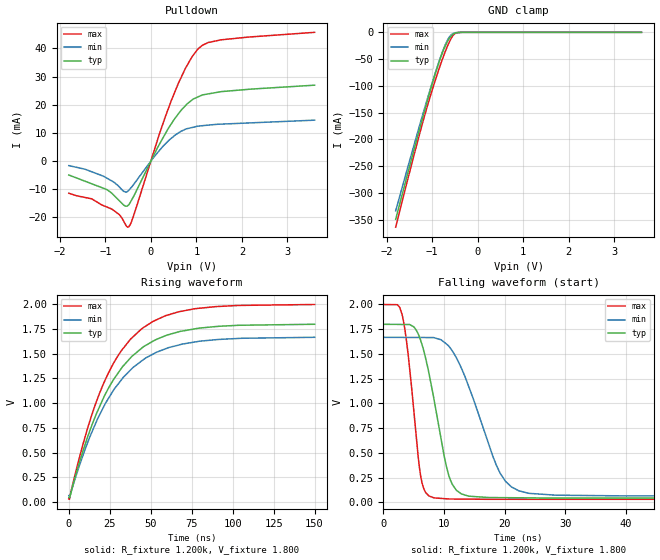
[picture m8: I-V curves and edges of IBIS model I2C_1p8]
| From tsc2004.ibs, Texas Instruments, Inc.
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| Model 1.8 V I2C
[Model]   I2C_1p8
Model_type   I/O_open_drain
Polarity   Non-Inverting
Enable   Active-Low
Vinl = 0.54
Vinh = 1.26
Vmeas = 0.9
Vref = 0.9
Cref = 15pF
Rref = 1200
|   typ   min   max
|   (nom PVT)   (Fast PVT)   (slow PVT)
|   Output High
C_comp   1.38702E-11   1.38702E-11   1.38702E-11
|   Output Low
|C_comp   1.34302E-11   1.32458E-11   1.39342E-11
| Where   nom PVT is  Nominal Process, 3.3V, 25C
|   Fast PVT is Strong Process, 3.6V, -40C
|   Slow PVT is Weak Process, 3.0V, 85C
|C_comp - from L-C Tank method, L = 1nH, peak frequency ~ 1.35GHz
[Model Spec]   | power 1.8, 1.65. 2 V
Vinl   0.54   0.495   0.6
Vinh   1.26   1.155   1.4
[Voltage Range]   1.8   1.65   2
[Temperature Range]   30   88   -40
|Ambient Temperature Range 27   85   -40
[Pullup Reference]   1.8   1.65   2
[Pulldown Reference]   0   0   0
[Power Clamp Reference]   1.8   1.65   2
[GND Clamp Reference]   0   0   0
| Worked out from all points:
|   slope of the pulldown table from 0 to 0.27 V, typ, clamps not added: 32.2 ohm
|   GND clamp passes 1 mA (typ) near -0.48 V on its own axis
|   falling waveform, R_fixture 1.200k, V_fixture 1.800: 20-80 % time 3.28ns typ, 5.65ns min, 1.95ns max; typ from 1.8 V to 0.044 V
|   rising waveform, R_fixture 1.200k, V_fixture 1.800: 20-80 % time 30.7ns typ, 31.5ns min, 29.5ns max; typ from 0.044 V to 1.8 V
[Pulldown]
|   Voltage   I(typ)   I(min)   I(max)
-1.8V     -4.973mA   -1.633mA   -11.46mA
-1.302V   -8.061mA   -3.786mA   -13.43mA
-858mV    -11.43mA   -7.078mA   -17.06mA
-601.5mV  -15.59mA   -10.74mA   -21.21mA
-489.1mV  -15.63mA   -10.47mA   -23.45mA
-383.6mV  -12.76mA   -8.464mA   -19.7mA
173.6mV   5.505mA    3.443mA    8.866mA
449.5mV   13.2mA     8.066mA    21.47mA
761.2mV   19.68mA    11.3mA     32.97mA
1.033V    22.76mA    12.38mA    39.77mA
1.544V    24.64mA    13.1mA     43.05mA
3.595V    26.94mA    14.51mA    45.72mA
[GND Clamp]
|   Voltage   I(typ)   I(min)   I(max)
-1.8V     -349.4mA   -333.7mA   -364.1mA
-1.542V   -265.7mA   -254.5mA   -277.1mA
-1.235V   -168mA     -162.2mA   -177.2mA
-1.103V   -127.5mA   -123.8mA   -137.2mA
-913.4mV  -72.53mA   -71.13mA   -85.05mA
-765mV    -35.94mA   -34.59mA   -48mA
-670.8mV  -18.24mA   -15.84mA   -27.36mA
-600mV    -8.634mA   -6.339mA   -14.15mA
-506.6mV  -1.685mA   -1.179mA   -2.932mA
-447.6mV  -559.6uA   -511.1uA   -577.9uA
-353.2mV  -32.62uA   -29.66uA   -19.2uA
3.595V    0A         0A         0A
[POWER Clamp]
|   SCR cell for ESD function. Effects occurr above VDD x 2
|   Voltage   I(typ)   I(min)   I(max)
-1.8V     0A         0A         0A
0V        0A         0A         0A
3.6V      0A         0A         0A
[Ramp]
R_load = 1200
|   typ   min   max
dV/dt_r   1.05295/3.05552e-008  0.951745/3.14117e-008   1.18078/2.93999e-008
dV/dt_f   1.05295/3.26932e-009  0.951745/5.63378e-009   1.18078/1.94029e-009
[Falling Waveform]
R_fixture = 1.200k
V_fixture = 1.800
V_fixture_min = 1.650
V_fixture_max = 2.000
C_fixture = 0.000
|  time   V(typ)   V(min)   V(max)
0s        1.799V     1.667V     1.999V
3.047ns   1.797V     1.667V     1.905V
4.061ns   1.797V     1.666V     1.504V
6.169ns   1.632V     1.666V     258.3mV
8.299ns   1.056V     1.665V     46.84mV
10.4ns    360.1mV    1.6V       36.48mV
12.01ns   124.2mV    1.463V     34.09mV
19.25ns   48.4mV     294.9mV    31.58mV
23.82ns   46.04mV    93.78mV    31.56mV
150ns     44.03mV    63.97mV    31.19mV
[Rising Waveform]
R_fixture = 1.200k
V_fixture = 1.800
V_fixture_min = 1.650
V_fixture_max = 2.000
C_fixture = 0.000
|  time   V(typ)   V(min)   V(max)
0s        44.03mV    63.97mV    31.19mV
813.1ps   61.83mV    65.7mV     63.43mV
5.279ns   333.1mV    308.2mV    374.4mV
11.47ns   656.4mV    599.3mV    746.4mV
21.16ns   1.053V     959.4mV    1.198V
31.59ns   1.341V     1.226V     1.52V
44.56ns   1.558V     1.429V     1.754V
59.26ns   1.685V     1.552V     1.887V
76.77ns   1.752V     1.619V     1.956V
150ns     1.799V     1.667V     1.999V
